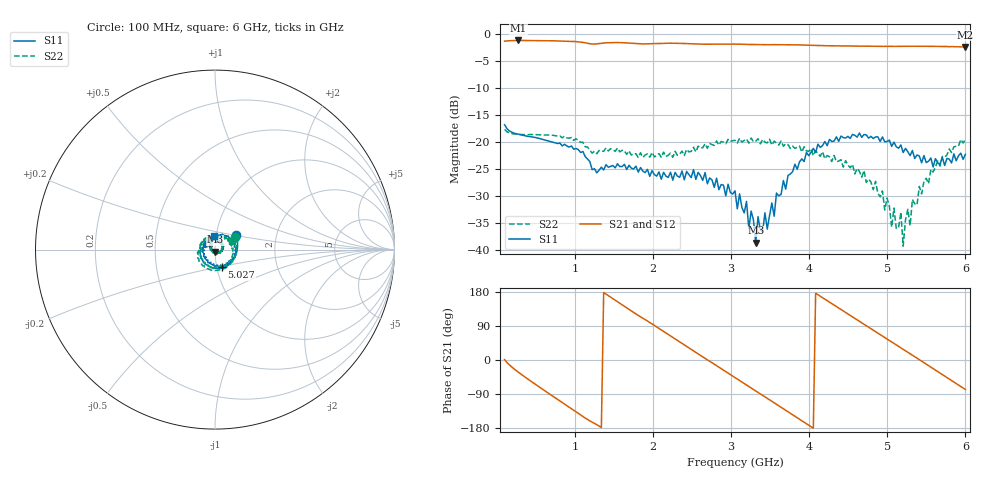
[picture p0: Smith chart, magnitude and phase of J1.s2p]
!Agilent Technologies,E8364B,MY43040379,A.07.50.67
!Agilent E8364B: A.07.50.67
!Date: Tuesday, March 24, 2026 10:35:05
!Correction: S11(Full 2 Port(1,2))
!S21(Full 2 Port(1,2))
!S12(Full 2 Port(1,2))
!S22(Full 2 Port(1,2))
!S2P File: Measurements: S11, S21, S12, S22:
# Hz S  dB  R 50
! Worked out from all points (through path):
!   201 points, 100 MHz to 6 GHz, reference 50 ohm
!   highest |S21| = -1.16 dB at 277 MHz (marker M1); lowest = -2.4 dB at 6 GHz (marker M2)
!   group delay of S21, straight-line fit = 370 ps
!   lowest |S11| = -38.7 dB at 3.316 GHz (marker M3), VSWR 1.02, Z = 49.9 - j1.16 ohm
!   |S11| at or under -10 dB: start of sweep to end of sweep
!   |S22| runs from -39.3 to -17.7 dB; largest |S21 - S12| = 0.004
!   S11 on the Smith chart (normalised r, x): 100 MHz: 1.25, +0.21; 5.027 GHz: 1.06, -0.21; 6 GHz: 0.98, +0.15
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1e8  -16.81 35.1  -1.30 0.9  -1.32 1.0  -17.66 32.2
2.77e8  -18.55 -23.4  -1.16 -32.3  -1.19 -32.5  -18.57 -24.7
6.9e8  -19.90 -100.6  -1.22 -91.7  -1.24 -91.7  -18.70 -99.0
1.103e9  -21.76 -179.4  -1.52 -149.2  -1.54 -149.2  -20.04 -170.3
1.5455e9  -24.04 134.3  -1.55 153.5  -1.57 153.6  -21.12 142.0
2.0765e9  -25.55 71.2  -1.70 83.4  -1.71 83.4  -22.15 83.3
2.578e9  -25.64 34.5  -1.83 16.0  -1.84 16.0  -20.76 40.3
3.05e9  -29.06 -32.8  -1.84 -46.6  -1.84 -46.6  -19.68 -25.9
3.1975e9  -31.01 -60.2  -1.88 -66.3  -1.90 -66.3  -19.45 -47.4
3.227e9  -36.11 -76.4  -1.91 -70.2  -1.91 -70.2  -20.21 -50.3
3.2565e9  -32.80 -64.4  -1.91 -74.0  -1.93 -74.0  -19.26 -53.9
3.3155e9  -38.69 -92.8  -1.94 -81.8  -1.95 -81.8  -19.85 -62.6
3.345e9  -33.84 -104.4  -1.93 -85.8  -1.95 -85.7  -19.38 -70.4
3.463e9  -36.15 174.6  -1.95 -101.2  -1.96 -101.3  -20.16 -87.9
3.64e9  -29.71 147.8  -1.93 -124.8  -1.96 -124.7  -19.84 -121.3
4.053e9  -21.18 69.2  -2.07 -180.0  -2.08 -179.9  -22.52 158.0
4.584e9  -18.75 -2.3  -2.20 110.1  -2.21 110.1  -25.92 52.8
5.0265e9  -19.65 -68.2  -2.25 51.9  -2.26 51.9  -31.91 -63.9
5.174e9  -20.54 -92.2  -2.25 32.4  -2.25 32.4  -33.02 -127.1
5.2035e9  -21.96 -95.6  -2.25 28.5  -2.27 28.5  -39.32 -156.1
5.41e9  -22.59 -140.2  -2.23 0.9  -2.25 0.9  -28.24 134.4
6e9  -22.29 93.8  -2.36 -77.9  -2.37 -77.8  -19.53 26.3
